FUNCTION_BLOCK FB_LN_IED_LD1_LEDGGIO1 EXTENDS FB_AcsiCommonLogicalNodeClass
VAR_INPUT
	NamPlt: FB_DO_IED_LD1_LEDGGIO1_NamPlt := (sClass:='LPL', bLinkResult:=THIS^.AddDataToContainer(ipData:=NamPlt));
	Beh: FB_DO_IED_LD1_LEDGGIO1_Beh := (sClass:='ENS', bLinkResult:=THIS^.AddDataToContainer(ipData:=Beh));
	Health: FB_DO_IED_LD1_LEDGGIO1_Health := (sClass:='ENS', bLinkResult:=THIS^.AddDataToContainer(ipData:=Health));
	Mod_: FB_DO_IED_LD1_LEDGGIO1_Mod := (sObjectName:='Mod', sClass:='ENC', bLinkResult:=THIS^.AddDataToContainer(ipData:=Mod_));
	AnOut1: FB_DO_IED_LD1_LEDGGIO1_AnOut1 := (sClass:='APC', bLinkResult:=THIS^.AddDataToContainer(ipData:=AnOut1));
	SPCSO1: FB_DO_IED_LD1_LEDGGIO1_SPCSO1 := (sClass:='SPC', bLinkResult:=THIS^.AddDataToContainer(ipData:=SPCSO1));
	DPCSO1: FB_DO_IED_LD1_LEDGGIO1_DPCSO1 := (sClass:='DPC', bLinkResult:=THIS^.AddDataToContainer(ipData:=DPCSO1));
	ISCSO1: FB_DO_IED_LD1_LEDGGIO1_ISCSO1 := (sClass:='INC', bLinkResult:=THIS^.AddDataToContainer(ipData:=ISCSO1));
END_VAR
VAR
END_VAR

END_FUNCTION_BLOCK
